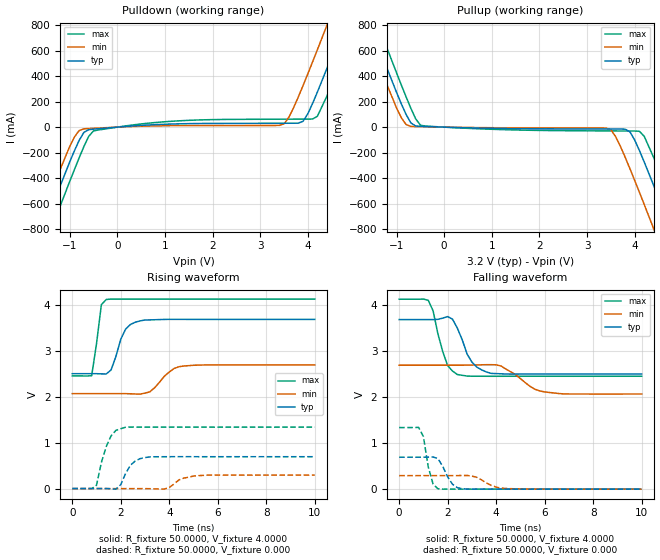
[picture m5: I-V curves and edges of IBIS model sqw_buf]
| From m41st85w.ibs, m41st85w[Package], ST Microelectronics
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|   Model sqw_buf
[Model]   sqw_buf
Model_type   Output
Polarity   Non-Inverting
Vmeas =   1.5000V
Cref =1.000e-10F
Rref =   0.6450k
Vref =   1.7300V
C_comp   3.8000pF   3.7000pF   3.9500pF
[Temperature Range]   27.0000   85.0000   -40.0000
[Voltage Range]   3.2000V   2.7000V   3.6000V
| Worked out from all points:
|   slope of the pulldown table from 0 to 0.48 V, typ, clamps not added: 36.6 ohm
|   slope of the pullup table from 0 to 0.48 V, typ, clamps not added: 94.9 ohm
|   rising waveform, R_fixture 50.0000, V_fixture 4.0000: 20-80 % time 471ps typ, 690ps min, 255ps max; typ from 2.51 V to 3.69 V
|   rising waveform, R_fixture 50.0000, V_fixture 0.000: 20-80 % time 457ps typ, 583ps min, 456ps max; typ from 0 V to 0.695 V
|   falling waveform, R_fixture 50.0000, V_fixture 4.0000: 20-80 % time 603ps typ, 991ps min, 499ps max; typ from 3.69 V to 2.51 V
|   falling waveform, R_fixture 50.0000, V_fixture 0.000: 20-80 % time 432ps typ, 637ps min, 292ps max; typ from 0.695 V to 0 V
[Pulldown]
| voltage   I(typ)   I(min)   I(max)
-3.2V     -2.415A    -2.266A    -2.589A
-1.6V     -843.1mA   -702.4mA   -1.009A
-1.4V     -650.1mA   -512.4mA   -813.1mA
-800mV    -103.1mA   -26.61mA   -239.7mA
-400mV    -12.67mA   -7.237mA   -22.25mA
3.4V      30.47mA    13.72mA    62.33mA
3.8V      31.28mA    236.8mA    62.81mA
4.2V      274.4mA    606.7mA    84.97mA
4.4V      459.7mA    798mA      242.5mA
4.8V      843.2mA    1.185A     619.7mA
5V        1.038A     1.381A     813.7mA
6.4V      2.415A     2.759A     2.192A
[Pullup]
| voltage   I(typ)   I(min)   I(max)
-3.2V     2.415A     2.265A     2.589A
-1.8V     1.037A     894.2mA    1.204A
-1.4V     649.4mA    511.6mA    812.4mA
-900mV    183.1mA    73.69mA    331mA
-500mV    6.248mA    3.443mA    15.4mA
3.4V      -14.64mA   -7.302mA   -29.56mA
3.9V      -37.07mA   -326mA     -30.29mA
4.1V      -184.1mA   -511.8mA   -32.64mA
4.4V      -459mA     -798mA     -239.6mA
4.8V      -842.9mA   -1.186A    -618.7mA
5V        -1.037A    -1.381A    -813mA
6.4V      -2.415A    -2.76A     -2.193A
[Ramp]
| variable   typ   min   max
dV/dt_r   1.4714/1.0097n   0.9466/2.0649n   1.8637/0.5543n
dV/dt_f   1.7403/0.5870n   1.3402/1.2910n   2.0485/0.2935n
R_load = 0.3330k
[Rising Waveform]
R_fixture = 50.0000
V_fixture = 4.0000
V_fixture_min = 2.7000
V_fixture_max = 5.5000
| time   V(typ)   V(min)   V(max)
0s        2.507V     2.072V     2.458V
800ps     2.507V     2.072V     2.463V
1.2ns     2.504V     2.072V     4.014V
1.4ns     2.502V     2.072V     4.127V
1.6ns     2.588V     2.072V     4.136V
2.2ns     3.482V     2.071V     4.136V
2.8ns     3.66V      2.062V     4.136V
3.2ns     3.682V     2.113V     4.136V
4.4ns     3.693V     2.66V      4.136V
10ns      3.692V     2.7V       4.136V
[Rising Waveform]
R_fixture = 50.0000
V_fixture = 0.000
V_fixture_min = 0.000
V_fixture_max = 0.000
| time   V(typ)   V(min)   V(max)
0s        1.378nV    1.573nV    1.077nV
1ns       21.15uV    1.554uV    74.68mV
1.2ns     287.4uV    100.8nV    569.5mV
1.6ns     -5.4mV     -4.481uV   1.149V
2ns       87.01mV    -5.712uV   1.307V
2.2ns     330.8mV    66.86uV    1.339V
2.6ns     603.8mV    278.7uV    1.342V
3.2ns     690.9mV    -3.203mV   1.341V
5.2ns     695.3mV    282mV      1.341V
10ns      695.2mV    293.9mV    1.341V
[Falling Waveform]
R_fixture = 50.0000
V_fixture = 4.0000
V_fixture_min = 2.7000
V_fixture_max = 5.5000
| time   V(typ)   V(min)   V(max)
0s        3.693V     2.7V       4.136V
1.2ns     3.692V     2.7V       4.113V
1.4ns     3.692V     2.7V       3.884V
1.6ns     3.699V     2.7V       3.379V
2ns       3.758V     2.7V       2.692V
2.4ns     3.506V     2.7V       2.496V
3ns       2.768V     2.702V     2.459V
3.8ns     2.52V      2.71V      2.458V
6ns       2.508V     2.117V     2.459V
10ns      2.507V     2.072V     2.458V
[Falling Waveform]
R_fixture = 50.0000
V_fixture = 0.000
V_fixture_min = 0.000
V_fixture_max = 0.000
| time   V(typ)   V(min)   V(max)
0s        695.3mV    293.9mV    1.341V
800ps     695.8mV    294mV      1.344V
1ns       695.9mV    294.1mV    1.146V
1.2ns     696.9mV    294.2mV    483.4mV
1.4ns     699.6mV    294.3mV    108mV
1.6ns     664.6mV    294.4mV    8.307mV
2.2ns     105.7mV    294.3mV    336.7uV
2.6ns     8.668mV    297.1mV    -626.8uV
4.4ns     13.89uV    13.59mV    -176.2uV
10ns      -11.69uV   -5.638uV   268.4uV
